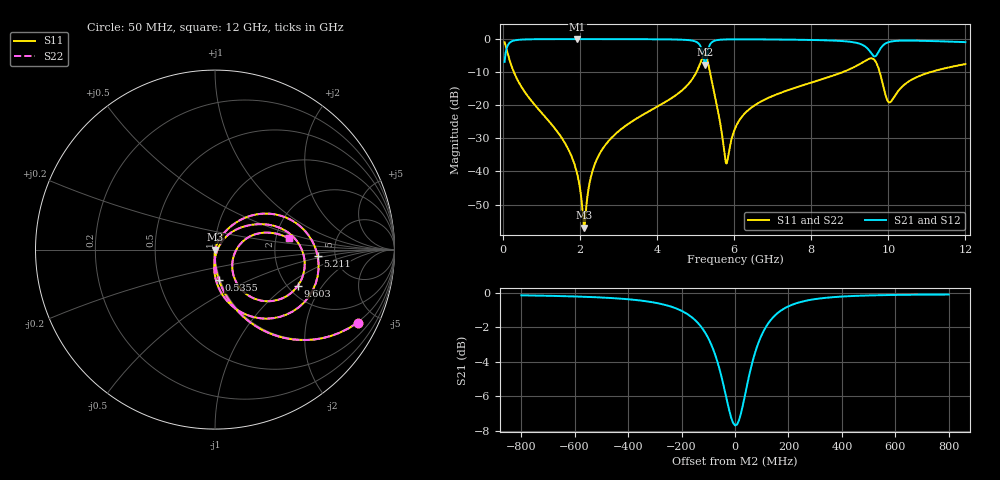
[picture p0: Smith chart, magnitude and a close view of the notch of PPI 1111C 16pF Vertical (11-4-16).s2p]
# GHz S MA R 50
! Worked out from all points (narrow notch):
!   1601 points, 50 MHz to 12 GHz, reference 50 ohm
!   highest |S21| = -0.01 dB at 1.94 GHz (marker M1); lowest = -7.7 dB at 5.248 GHz (marker M2)
!   notch at M2: 7.5 dB deep, 133 MHz wide at half that depth
!   lowest |S11| = -57.0 dB at 2.111 GHz (marker M3), VSWR 1.00, Z = 50.1 - j0.0434 ohm
!   |S11| at or under -10 dB: 291.3 MHz to 5.024 GHz (4.733 GHz wide, 178 % of centre); 5.375 GHz to 8.818 GHz (3.442 GHz wide, 48.5 % of centre); 9.777 GHz to 11.09 GHz (1.316 GHz wide, 12.6 % of centre)
!   |S22| runs from -57.0 to -1.0 dB; largest |S21 - S12| = 0
!   S11 on the Smith chart (normalised r, x): 50 MHz: 0.98, -3.92; 535.5 MHz: 0.99, -0.34; 5.211 GHz: 3.64, -0.39; 9.603 GHz: 2.26, -1.22; 12 GHz: 2.37, +0.36
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0.05  0.8922 -27.1  0.4515 62.9  0.4515 62.9  0.8922 -27.1
0.2217813  0.4035 -67.3  0.9145 22.7  0.9145 22.7  0.4035 -67.3
0.5354688  0.171 -82.6  0.9845 7.1  0.9845 7.1  0.171 -82.6
1.566156  0.02986 -93.9  0.9983 -6.2  0.9983 -6.2  0.02986 -93.9
1.939594  0.008809 -90.5  0.9985 -9.3  0.9985 -9.3  0.008809 -90.5
2.044156  0.003718 -78.3  0.9985 -10.1  0.9985 -10.1  0.003718 -78.3
2.111375  0.001414 -17.8  0.9985 -10.6  0.9985 -10.6  0.001414 -17.8
2.3205  0.009751 69.0  0.9983 -12.2  0.9983 -12.2  0.009751 69.0
2.604312  0.02248 71.6  0.998 -14.4  0.998 -14.4  0.02248 71.6
4.038312  0.09739 62.5  0.992 -25.7  0.992 -25.7  0.09739 62.5
5.061531  0.3519 34.8  0.877 -45.3  0.877 -45.3  0.3519 34.8
5.210906  0.5729 -3.6  0.5162 -50.4  0.5162 -50.4  0.5729 -3.6
5.24825  0.5901 -22.5  0.4122 -30.8  0.4122 -30.8  0.5901 -22.5
5.4275  0.2236 -83.7  0.8973 -14.7  0.8973 -14.7  0.2236 -83.7
5.786  0.01376 -36.9  0.9861 -28.3  0.9861 -28.3  0.01376 -36.9
6.025  0.04435 47.0  0.9903 -32.1  0.9903 -32.1  0.04435 47.0
6.600094  0.1055 48.8  0.9887 -38.3  0.9887 -38.3  0.1055 48.8
8.019156  0.221 36.9  0.9682 -51.4  0.9682 -51.4  0.221 36.9
9.199219  0.3998 15.9  0.8694 -67.2  0.8694 -67.2  0.3998 15.9
9.602531  0.5037 -23.5  0.5648 -65.0  0.5648 -65.0  0.5037 -23.5
10.01331  0.1108 -22.7  0.8999 -50.2  0.8999 -50.2  0.1108 -22.7
12  0.4187 8.6  0.8978 -80.0  0.8978 -80.0  0.4187 8.6
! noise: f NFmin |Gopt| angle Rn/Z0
0.05  0.0003764  0.8699  1.376  0.0006227
1.372  0.003846  0.6806  7.099  0.002321
2.701  0.006557  0.6427  13.39  0.003425
4.031  0.01075  0.6734  19.63  0.006164
5.36  0.09904  0.9462  26.48  0.3908
6.682  0.01775  0.6838  32.13  0.01008
8.012  0.02177  0.6971  37.75  0.01262
9.341  0.09092  0.9077  44.25  0.1858
10.67  0.04394  0.8008  49.57  0.0378
12  0.03203  0.7185  53.79  0.01803
